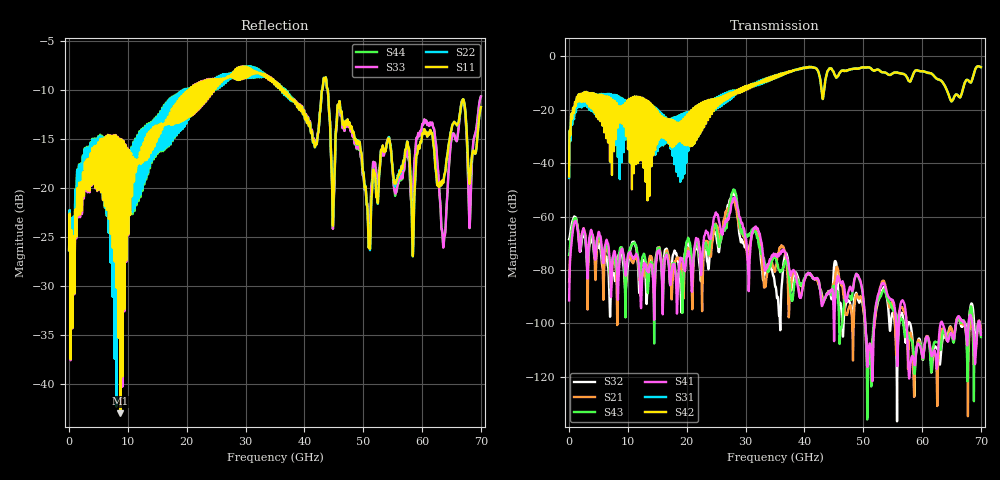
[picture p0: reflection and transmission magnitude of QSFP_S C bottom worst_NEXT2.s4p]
! AWR Design Environment (8415) Tue Jan 08 12:52:55 2019
! Document = 'QSFP Channel_S'
! nPorts: 4, nXvals: 7001
# HZ S DB R 50
!Freq DBS11 AngS11 DBS12 AngS12 DBS13 AngS13 DBS14 AngS14
!	DBS21 AngS21 DBS22 AngS22 DBS23 AngS23 DBS24 AngS24
!	DBS31 AngS31 DBS32 AngS32 DBS33 AngS33 DBS34 AngS34
!	DBS41 AngS41 DBS42 AngS42 DBS43 AngS43 DBS44 AngS44
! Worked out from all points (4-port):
!   7000 points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, 10 MHz to 70 GHz, reference 50 ohm
!   strongest paths, dB at 10 MHz, 17.51 GHz, 35.01 GHz, 52.51 GHz, 70 GHz:
!     S42: -45.0, -33.1, -7.3, -5.0, -4.0
!     S31: -45.5, -26.4, -7.4, -5.0, -4.0
!     S41: -91.4, -79.4, -74.4, -89.4, -104.3
!     S43: -74.4, -78.7, -75.3, -91.0, -105.1
!     S21: -84.3, -88.0, -80.5, -90.2, -102.1
!     S32: -68.5, -76.7, -85.9, -91.8, -103.3
!   lowest |S11| = -43.0 dB at 8.74 GHz (marker M1), VSWR 1.01, Z = 50.7 + j0.249 ohm
!   |S11| at or under -10 dB: start of sweep to 20.44 GHz; 36.44 GHz to 43.03 GHz (6.585 GHz wide, 16.6 % of centre); 43.97 GHz to end of sweep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
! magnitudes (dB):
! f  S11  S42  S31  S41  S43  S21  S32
! 10 MHz  -26.4  -45.0  -45.5  -91.4  -74.4  -84.3  -68.5
! 1.64 GHz  -20.4  -14.2  -15.6  -69.2  -68.2  -67.5  -68.2
! 8.74 GHz  -43.0  -20.4  -16.2  -73.4  -71.6  -73.0  -73.0
! 22.42 GHz  -9.3  -17.7  -18.9  -81.8  -80.6  -78.0  -83.5
! 27.99 GHz  -8.3  -14.4  -14.7  -53.2  -49.9  -54.2  -51.4
! 33.77 GHz  -8.8  -9.2  -9.4  -77.9  -80.4  -79.5  -77.9
! 70 GHz  -11.8  -4.0  -4.0  -104.3  -105.1  -102.1  -103.3
